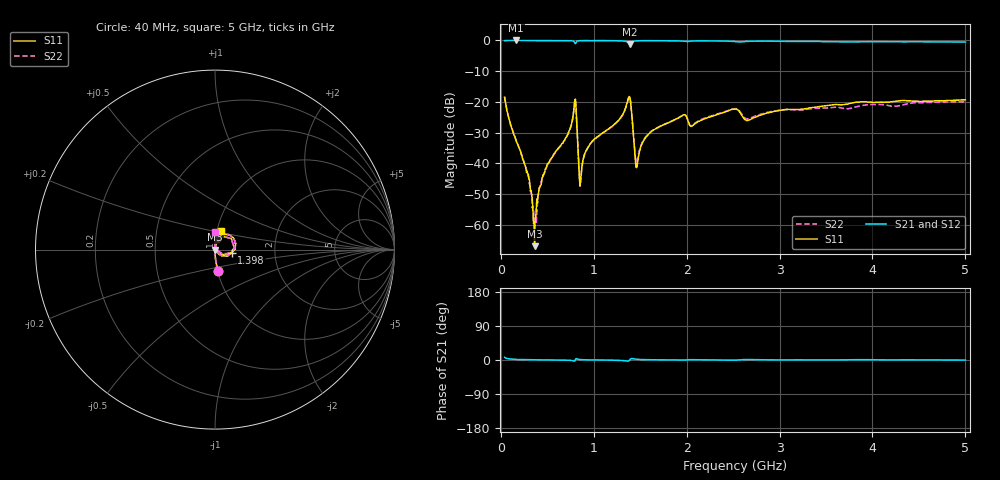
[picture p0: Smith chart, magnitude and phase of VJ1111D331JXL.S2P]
! VJ1111D331JXL
! DATE 02/15/2022  13:39
! CAPACITORS MOUNTED IN SERIES ON 25 MIL THICK MICROSTRIP SUBSTRATE
# GHz  S  MA  R  50.00
!  FREQ  S11M  S11A  S21M  S21A  S12M  S12A  S22M  S22A
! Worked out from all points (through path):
!   801 points, 40 MHz to 5 GHz, reference 50 ohm
!   highest |S21| = 0.00 dB at 164 MHz (marker M1); lowest = -1.1 dB at 1.385 GHz (marker M2)
!   lowest |S11| = -67.0 dB at 362.4 MHz (marker M3), VSWR 1.00, Z = 50 - j0.00357 ohm
!   |S11| at or under -10 dB: start of sweep to end of sweep
!   |S22| runs from -59.3 to -18.4 dB; largest |S21 - S12| = 0.011
!   S11 on the Smith chart (normalised r, x): 40 MHz: 1.00, -0.24; 1.398 GHz: 1.21, -0.04; 5 GHz: 1.04, +0.22
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0.04  0.1187 -82.1  0.9931 6.7  0.9932 6.9  0.1206 -82.5
0.164  0.02344 -85.9  1 1.6  0.9964 1.7  0.02359 -87.0
0.288  0.006863 -81.8  0.9972 0.8  0.9999 0.8  0.006933 -80.2
0.3624  0.0004485 -4.6  0.9954 0.5  1.001 0.5  0.001203 -27.3
0.474  0.007563 85.3  0.9975 0.2  0.9989 0.4  0.007377 85.4
0.7158  0.02898 83.2  0.9942 -0.5  0.9972 -0.6  0.02845 84.4
0.784  0.07145 65.1  0.9667 -2.6  0.9724 -2.6  0.07112 66.6
0.8088  0.07932 -27.8  0.9262 3.6  0.931 3.6  0.07843 -26.2
0.846  0.005416 -18.3  0.9903 1.4  0.9956 1.4  0.005891 -19.3
0.8708  0.008324 69.8  0.993 0.9  0.9983 0.9  0.008262 72.0
0.9576  0.02042 84.3  0.9932 0.3  0.9996 0.3  0.02012 86.8
1.3854  0.1216 17.3  0.8801 -0.2  0.8852 -0.2  0.1193 21.9
1.3978  0.09523 -11.0  0.902 3.3  0.9072 3.2  0.09365 -5.9
1.4412  0.01454 -25.1  0.9792 2.6  0.9848 2.5  0.01561 -12.9
1.466  0.0089 47.4  0.9862 1.9  0.9919 1.9  0.01104 48.1
1.5466  0.02486 84.6  0.9909 1.0  0.9945 0.9  0.02555 84.6
1.6954  0.03839 86.8  0.9891 0.5  0.9944 0.4  0.03876 87.8
2.52  0.07632 70.2  0.9604 -0.4  0.9658 -0.4  0.07759 76.5
2.6564  0.04988 71.6  0.9671 1.3  0.9725 1.1  0.05303 77.3
3.3508  0.08106 81.3  0.9633 0.3  0.9687 0.1  0.0778 89.9
4.1754  0.09941 75.3  0.9525 0.3  0.96 0.1  0.08692 88.9
5  0.1081 73.4  0.9426 -0.1  0.9478 -0.4  0.1008 88.6
